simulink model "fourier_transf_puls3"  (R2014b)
settings: Solver=ode45  StartTime=0.0  StopTime=10.0  RelTol=1e-3
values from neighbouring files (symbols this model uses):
  N = 4*1024    (= 4096)    [ad_test_12.m]    (also in ad_test_2.m; ad_test_3.m; DA_wandler_spektr_1.m = 1000; DA_wandler_spektr_2.m = 1024)
  Ts = 1/fs    (= 0.00025)    [abtast_rate_1.m]    (also in ad_test_12.m = 0.0009765625; ad_test_2.m = 0.00048828125; ad_test_3.m = 0.00048828125; DA_wandler_spektr_1.m = 0.01)
  w = hanning(N)    [fenster.m]    (also in fourier_transf_puls_3.m = ones(1,N); fourier_transf_puls_4.m = ones(1,N); anti_alias_1.m = sum(hann(nfft).^2)/nfft; anti_alias_2.m = sum(hann(nfft).^2)/nfft)
  wf = sqrt(N/sum(w.^2))    [fourier_transf_puls_3.m]    (also in fourier_transf_puls_4.m)
undefined symbols (not defined in the file or in its folder): get
libraries: dspxfrm3 x1, simulink x1, dspsnks4 x1

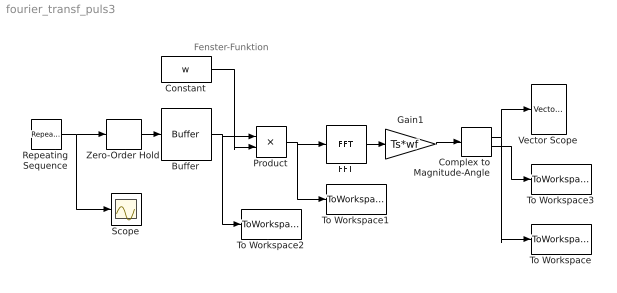
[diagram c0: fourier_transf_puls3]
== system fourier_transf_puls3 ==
  note: Fenster-Funktion
  Buffer : Buffer  N=N  TreatMby1Signals=One channel
  Complex to Magnitude-Angle : ComplexToMagnitudeAngle
  Constant : Constant  Value=w
  FFT : dspxfrm3/FFT  CompMethod=Table lookup  TableOpt=NEW  TableOptActive=Speed  BitRevOrder=off  InheritFFTLength=on  FFTLength=64  WrapInput=on  RowConvenienceOn=on  FFTImplementation=Auto  SkipNorm=off  firstCoeffDataTypeStr=Inherit: Same word length as input  firstCoeffLastDataTypeStr=Inherit: Same word length as input  outputMin=[]  outputMax=[]  roundingMode=Floor  overflowMode=off
  Gain1 : Gain  Gain=Ts*wf
  Product : Product
  Repeating Sequence : simulink/Sources/Repeating Sequence  rep_seq_t=t  rep_seq_y=yi
  Scope : Scope
  To Workspace : ToWorkspace  VariableName=y  SaveFormat=Structure  SampleTime=-1
  To Workspace1 : ToWorkspace  VariableName=y1  SaveFormat=Structure  SampleTime=-1
  To Workspace2 : ToWorkspace  VariableName=y2  SaveFormat=Structure  SampleTime=-1
  To Workspace3 : ToWorkspace  VariableName=y3  SaveFormat=Structure  SampleTime=-1
  Vector Scope : dspsnks4/Vector Scope  ScopeProperties=on  Domain=Frequency  HorizSpan=1  DisplayProperties=off  AxisGrid=on  Memory=off  FrameNumber=on  AxisLegend=off  AxisZoom=off  OpenScopeAtSimStart=on  OpenScopeImmediately=off  FigPos=get(0,'defaultfigureposition')  AxisProperties=off  XUnits=Hertz  XRange=[0...Fs]  InheritXIncr=off  XIncr=1/1024  XLabel=Time  XLimit=User-defined  XMin=1.0667  XMax=1022.9333  XStart=0  YUnits=dB  YLabel=dB  LineProperties=off  XAxisParamsVer=6.9
  Zero-Order Hold : ZeroOrderHold  SampleTime=Ts
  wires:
  Repeating Sequence/1 -> Scope/1, Zero-Order Hold/1
  Zero-Order Hold/1 -> Buffer/1
  Complex to Magnitude-Angle/1 -> To Workspace/1, Vector Scope/1
  Complex to Magnitude-Angle/2 -> To Workspace3/1
  Buffer/1 -> To Workspace2/1, Product/1
  FFT/1 -> Gain1/1
  Constant/1 -> Product/2
  Product/1 -> To Workspace1/1, FFT/1
  Gain1/1 -> Complex to Magnitude-Angle/1
